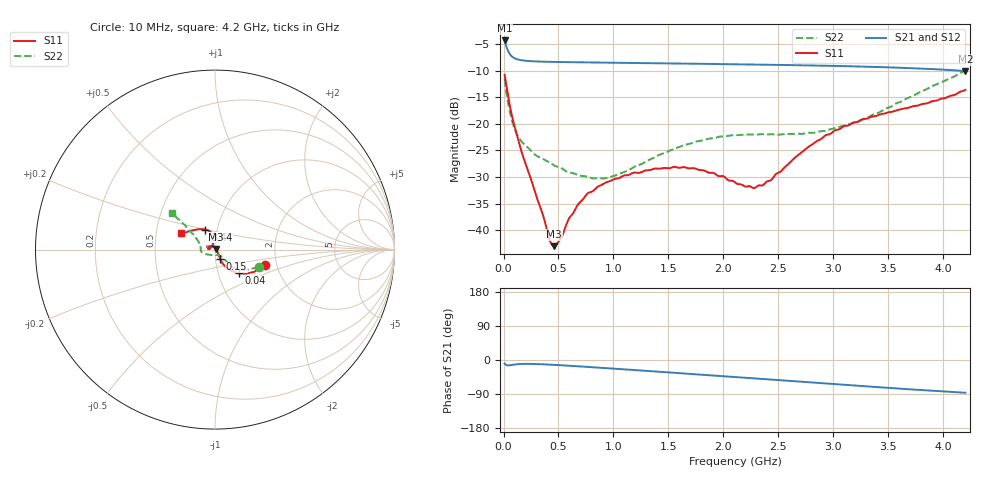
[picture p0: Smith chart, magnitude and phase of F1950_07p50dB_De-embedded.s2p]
! Integrated Device Technology
! Corporate Headquarters
! 6024 Silver Creek Valley Road
! San Jose, CA 95138  USA
! Phone:  1-408-284-8200
! Toll Free:  1-800-223-1366
! Webpage:  http://www.idt.com/
! Timing and RF Division
! 515 Groton Road, Suite 102
! Westford, MA 01886-6024
! Device:  F1950
! Description: 7-bit 0.25 dB Digital Step Attenuator
! Frequency:  150.0 -  4000.00 MHz
! Package:  4x4 mm Thin QFN Plastic Package: 24 pin
! Ports:  2 RF, 12 DC
!  Pin  1  = D0
!  Pin  2  = VDD
!  Pin  3  = Vmode
!  Pin  4  = GND
!  Pin  5  = RF1  =  Port 1
!  Pin  6  = GND
!  Pin  7  = GND
!  Pin  8  = GND
!  Pin  9  = GND
!  Pin 10  = GND
!  Pin 11  = GND
!  Pin 12  = GND
!  Pin 13  = GND
!  Pin 14  = RF2  =  Port 2
!  Pin 15  = GND
!  Pin 16  = LE
!  Pin 17  = CLK
!  Pin 18  = DATE
!  Pin 19  = D6
!  Pin 20  = D5
!  Pin 21  = D4
!  Pin 22  = D3
!  Pin 23  = D2
!  Pin 24  = D1
! State:  30
! Atten State:  7.50 dB
! Voltage:  +5.00 Volts
! Current:  Not Measured mA
! Data:  The device was measured on a the F195X evaluation board which has
!  individual transmission lines to the RF pins.  Data was collected
!  using a calibrated network analyzer.  The evaluation board was
!  de-embedded using a TRL calibration technique.
!  The reference plane is the edge of the package pin.
! Misc:  Board 2019
!  Action Tracker AT0250
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# GHz S dB R 50
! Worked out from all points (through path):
!   420 points, 10 MHz to 4.2 GHz, reference 50 ohm
!   highest |S21| = -4.33 dB at 10 MHz (marker M1); lowest = -10.1 dB at 4.2 GHz (marker M2)
!   group delay of S21, straight-line fit = 54.3 ps
!   lowest |S11| = -43.0 dB at 460 MHz (marker M3), VSWR 1.01, Z = 50.6 + j0.345 ohm
!   |S11| at or under -10 dB: start of sweep to end of sweep
!   |S22| runs from -30.3 to -10.0 dB; largest |S21 - S12| = 0.0005
!   S11 on the Smith chart (normalised r, x): 10 MHz: 1.72, -0.32; 40 MHz: 1.26, -0.34; 150 MHz: 1.05, -0.11; 3.44 GHz: 0.88, +0.20; 4.2 GHz: 0.67, +0.13
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0.01  -10.78 -17.2  -4.33 -9.1  -4.33 -9.1  -11.64 -21.8
0.04  -14.53 -44.5  -6.23 -14.4  -6.23 -14.4  -15.93 -41.7
0.09  -19.65 -59.5  -7.55 -12.4  -7.55 -12.4  -20.28 -45.8
0.15  -24.27 -61.3  -8.00 -10.6  -8.00 -10.6  -22.93 -46.0
0.29  -33.06 -48.5  -8.27 -10.6  -8.27 -10.6  -25.85 -47.5
0.42  -41.83 -4.2  -8.35 -12.2  -8.35 -12.2  -27.30 -50.6
0.46  -43.01 28.8  -8.37 -12.8  -8.36 -12.8  -27.84 -53.3
0.51  -41.89 66.7  -8.38 -13.6  -8.38 -13.6  -28.18 -56.2
0.59  -38.05 95.5  -8.41 -15.0  -8.41 -15.0  -29.11 -61.5
0.71  -34.48 113.9  -8.44 -17.2  -8.44 -17.2  -29.79 -72.7
0.77  -32.99 119.1  -8.46 -18.4  -8.46 -18.4  -30.03 -78.9
0.96  -30.82 134.3  -8.51 -22.0  -8.51 -22.0  -30.06 -104.2
1.41  -28.43 163.4  -8.62 -30.9  -8.62 -30.9  -25.89 -147.6
1.74  -28.38 175.4  -8.70 -37.5  -8.70 -37.5  -23.40 -162.4
2.11  -31.09 166.0  -8.81 -45.1  -8.81 -45.1  -22.15 -173.0
2.27  -32.08 143.5  -8.86 -48.3  -8.85 -48.3  -22.03 -176.7
2.36  -31.53 128.5  -8.89 -50.1  -8.89 -50.2  -21.94 -179.0
2.81  -23.85 97.0  -9.03 -59.4  -9.03 -59.4  -21.71 166.8
3.09  -20.50 101.8  -9.15 -65.2  -9.15 -65.2  -20.40 157.7
3.44  -18.17 115.5  -9.35 -72.3  -9.34 -72.4  -17.57 146.9
3.51  -17.79 118.4  -9.39 -73.7  -9.38 -73.8  -16.91 145.8
4.2  -13.61 154.0  -10.09 -86.4  -10.09 -86.4  -10.00 139.7
